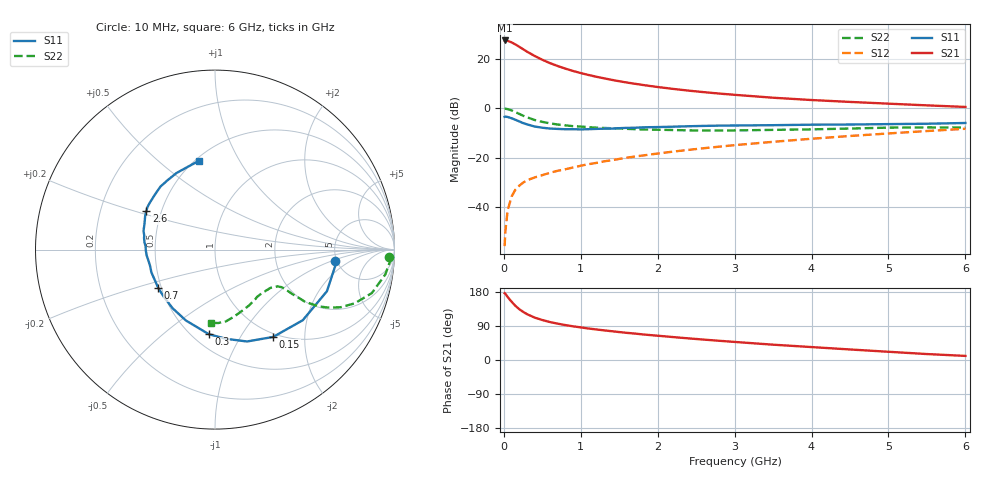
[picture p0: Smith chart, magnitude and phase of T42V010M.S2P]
! Infineon Technologies  Discrete & RF Semiconductors
! BFR182T
! Si NPN RF Bipolar Junction Transistor in SC75
! VCE = 2 V  IC = 10 mA
! Common Emitter S-Parameters:  October  1999
# GHz  S  MA  R  50
!  f  S11  S21  S12  S22
! GHz  MAG  ANG  MAG  ANG  MAG  ANG  MAG  ANG
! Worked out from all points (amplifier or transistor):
!   36 points, 10 MHz to 6 GHz, reference 50 ohm
!   highest |S21| = 27.5 dB at 10 MHz (marker M1)
!   |S21| within 3 dB of that: start of sweep to 222.5 MHz
!   unconditionally stable (mu >= 1): 919.1 MHz to 3.804 GHz
!   at 250 MHz: K = 0.47, MSG = 27.1 dB, |S12| = -30.2 dB
!   at 1.4 GHz: K = 1.09, MAG = 14.5 dB, |S12| = -21.1 dB
!   at 6 GHz: K = 0.84, MSG = 4.4 dB, |S12| = -8.3 dB
!   lowest NFmin = 1.50 dB at 450 MHz
!   S11 on the Smith chart (normalised r, x): 10 MHz: 4.82, -1.09; 150 MHz: 0.95, -1.40; 300 MHz: 0.60, -0.73; 700 MHz: 0.48, -0.24; 2.6 GHz: 0.41, +0.22; 6 GHz: 0.52, +0.69
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0.01  0.6709 -5.3  23.7 176.3  0.0016 87.4  0.9716 -2.4
0.02  0.6782 -6.8  23.69 174.6  0.0032 90.1  0.9795 -3.4
0.05  0.6653 -20.4  23.26 166.2  0.0086 84.9  0.9592 -8.3
0.1  0.6277 -38.8  21.68 154.0  0.0161 75.0  0.9067 -15.5
0.15  0.5847 -56.3  19.68 143.0  0.0224 68.6  0.8346 -21.0
0.2  0.5421 -70.8  17.67 134.2  0.0269 63.9  0.7692 -24.7
0.25  0.5014 -82.7  15.75 127.1  0.031 60.2  0.7067 -27.2
0.3  0.4729 -94.1  14.09 121.2  0.0346 58.9  0.6583 -28.7
0.4  0.427 -112.3  11.51 111.9  0.0396 58.0  0.5785 -30.1
0.5  0.4031 -125.9  9.629 105.5  0.0441 58.2  0.5299 -29.9
0.6  0.3881 -137.2  8.221 100.1  0.0492 58.5  0.4948 -29.9
0.7  0.3815 -146.0  7.188 95.9  0.054 59.7  0.4679 -29.6
0.9  0.3764 -160.5  5.703 88.9  0.063 62.1  0.4337 -29.4
1.1  0.3764 -171.1  4.735 83.1  0.0736 63.6  0.4146 -30.0
1.3  0.3858 -179.4  4.053 78.2  0.0837 64.6  0.3984 -31.2
1.6  0.4006 170.7  3.323 71.6  0.0996 65.6  0.3823 -33.4
2.2  0.423 157.7  2.47 60.5  0.1321 66.4  0.3622 -40.2
2.6  0.439 150.8  2.122 53.8  0.1549 66.0  0.3541 -45.5
3.5  0.4541 137.3  1.636 40.4  0.2088 63.6  0.3645 -58.6
4.5  0.4682 124.3  1.345 27.8  0.2742 59.2  0.388 -74.1
5.5  0.4858 108.0  1.145 15.7  0.3454 53.3  0.4095 -87.5
6  0.5029 100.1  1.064 10.8  0.3834 49.6  0.4085 -93.1
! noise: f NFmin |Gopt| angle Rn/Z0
0.45  1.5  0.26  43  0.28
0.9  1.6  0.24  87  0.22
1.8  2.1  0.2  170  0.2
